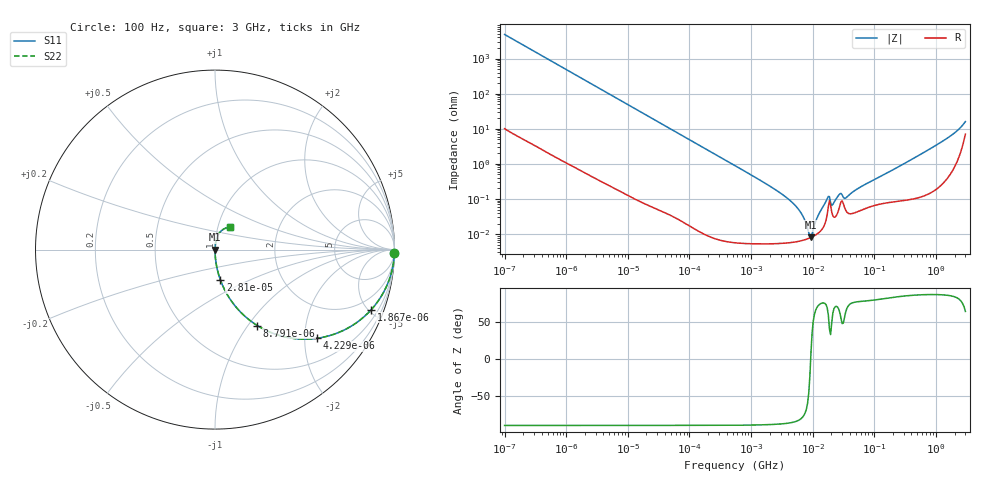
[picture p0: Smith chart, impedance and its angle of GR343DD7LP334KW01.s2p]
!Murata Part Number: GR343DD7LP334KW01
!These Parameters are Measured in Series Mode Connection
!Data Generated on Mar 13, 2026
!  o--ll--o
!Port1  Port2
!  o------o
!Operation Temp=25[degC], DC Bias Voltage=0[V]
!Freq. Start=100[Hz] Stop=3[GHz] 401[Steps]
# Hz S RI R 50
!Freq.(Hz) S11(Real) S11(Imag) S21(Real) S21(Imag) S12(Real) S12(Imag) S22(Real) S22(Imag)
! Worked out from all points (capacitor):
!   401 points, 100 Hz to 3 GHz, reference 50 ohm
!   read as one part in series: C = 329 nF near 109 Hz
!   lowest |Z| = 8.15 mohm at 9.382 MHz (marker M1)
!   series resonance near 9.263 MHz, so ESL is about 900 pH
!   S11 on the Smith chart (normalised r, x): 100 Hz: 1, -97; 1.867 kHz: 1.01, -5.21; 4.229 kHz: 1.01, -2.30; 8.791 kHz: 1.00, -1.11; 28.1 kHz: 1.00, -0.35; 3 GHz: 1.14, +0.29
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100  0.9995 -0.0206  0.000469 0.0206  0.000469 0.0206  0.9995 -0.0206
536  0.9877 -0.109  0.0123 0.109  0.0123 0.109  0.9877 -0.109
1788  0.8802 -0.3235  0.1198 0.3235  0.1198 0.3235  0.8802 -0.3235
1867  0.8709 -0.3342  0.1291 0.3342  0.1291 0.3342  0.8709 -0.3342
4229  0.5696 -0.4939  0.4304 0.4939  0.4304 0.4939  0.5696 -0.4939
8791  0.2356 -0.4231  0.7644 0.4231  0.7644 0.4231  0.2356 -0.4231
28103  0.0298 -0.1684  0.9702 0.1684  0.9702 0.1684  0.0298 -0.1684
31977  0.0232 -0.1491  0.9768 0.1491  0.9768 0.1491  0.0232 -0.1491
547723  0.000136 -0.00892  0.9999 0.00892  0.9999 0.00892  0.000136 -0.00892
4323298  5.79e-05 -0.000892  0.9999 0.000892  0.9999 0.000892  5.79e-05 -0.000892
6368694  6.42e-05 -0.000411  0.9999 0.000411  0.9999 0.000411  6.42e-05 -0.000411
8607956  7.54e-05 -7.98e-05  0.9999 7.98e-05  0.9999 7.98e-05  7.54e-05 -7.98e-05
9381788  8.03e-05 1.41e-05  0.9999 -1.41e-05  0.9999 -1.41e-05  8.03e-05 1.41e-05
9794414  8.32e-05 6.15e-05  0.9999 -6.15e-05  0.9999 -6.15e-05  8.32e-05 6.15e-05
1.214626e7  0.000105 0.000313  0.9999 -0.000313  0.9999 -0.000313  0.000105 0.000313
1.713898e7  0.000354 0.00094  0.9996 -0.00094  0.9996 -0.00094  0.000354 0.00094
2.12544e7  0.000328 0.000626  0.9997 -0.000626  0.9997 -0.000626  0.000328 0.000626
2.751729e7  0.00065 0.00124  0.9993 -0.00124  0.9993 -0.00124  0.00065 0.00124
3.562563e7  0.000428 0.00104  0.9996 -0.00104  0.9996 -0.00104  0.000428 0.00104
1.751444e8  0.00083 0.00592  0.9992 -0.00592  0.9992 -0.00592  0.00083 0.00592
1.324213e9  0.00494 0.0455  0.9951 -0.0455  0.9951 -0.0455  0.00494 0.0455
3e9  0.0818 0.1236  0.9182 -0.1236  0.9182 -0.1236  0.0818 0.1236
